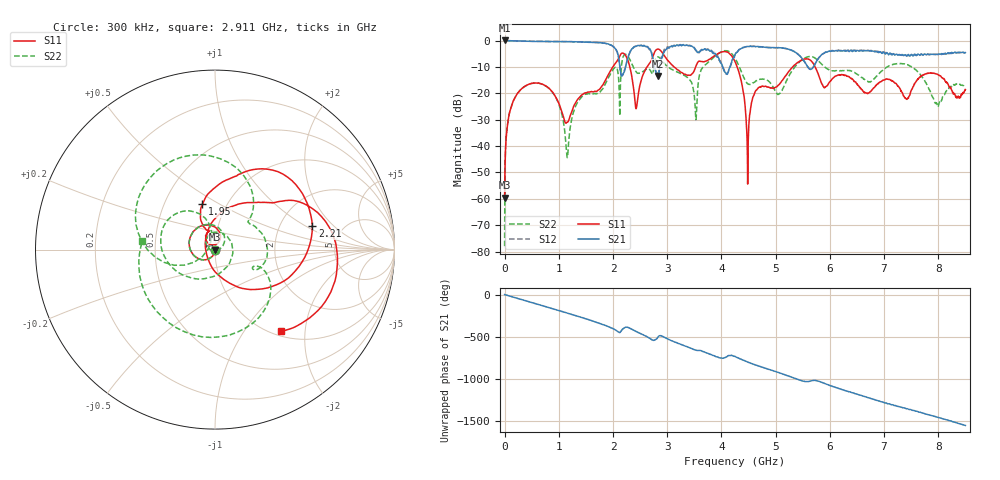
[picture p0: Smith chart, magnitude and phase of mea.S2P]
!Agilent Technologies,E5071B,MY42402595,A.08.01
!Date: Mon Jan 01 22:53:59 2001
!Data & Calibration Information:
!Freq	S11:SOLT2(ON)	S21:SOLT2(ON)	S12:SOLT2(ON)	S22:SOLT2(ON)
# Hz S dB R 50
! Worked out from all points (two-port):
!   1601 points, 300 kHz to 8.5 GHz, reference 50 ohm
!   highest |S21| = 0.04 dB at 300 kHz (marker M1); lowest = -13.5 dB at 2.821 GHz (marker M2)
!   |S21| within 3 dB of the highest: start of sweep to 2.038 GHz; 4.368 GHz to 5.173 GHz (804.4 MHz wide, 16.9 % of centre)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
!   lowest |S11| = -59.6 dB at 300 kHz (marker M3), VSWR 1.00, Z = 50 - j0.101 ohm
!   |S11| at or under -10 dB: start of sweep to 1.997 GHz; 4.291 GHz to 5.313 GHz (1.022 GHz wide, 21.3 % of centre); 5.728 GHz to end of sweep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
!   |S22| runs from -78.0 to -3.8 dB; largest |S21 - S12| = 0.071
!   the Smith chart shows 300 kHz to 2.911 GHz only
!   S11 on the Smith chart (normalised r, x): 300 kHz: 1.00, -0.00; 1.95 GHz: 0.77, +0.42; 2.21 GHz: 3.04, +1.15; 2.911 GHz: 1.09, -1.50
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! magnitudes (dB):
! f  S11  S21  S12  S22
! 300 kHz  -59.6  0.0  0.0  -78.0
! 64.05 MHz  -30.4  0.0  0.0  -30.4
! 250 MHz  -19.7  -0.1  -0.1  -19.8
! 845 MHz  -18.6  -0.4  -0.4  -18.7
! 1.153 GHz  -30.9  -0.4  -0.4  -44.3
! 1.419 GHz  -20.7  -0.5  -0.6  -21.4
! 1.95 GHz  -11.6  -1.6  -1.7  -12.7
! 2.21 GHz  -5.1  -11.7  -11.2  -5.4
! 2.433 GHz  -25.3  -2.1  -2.0  -12.0
! 2.821 GHz  -3.3  -13.5  -12.4  -6.2
! 2.837 GHz  -3.2  -12.7  -12.2  -6.2
! 2.911 GHz  -4.7  -5.7  -6.3  -7.8
! 3.522 GHz  -10.1  -3.4  -3.7  -28.2
! 3.676 GHz  -8.1  -3.3  -3.2  -9.7
! 4.25 GHz  -7.9  -5.3  -5.5  -6.7
! 4.489 GHz  -45.0  -2.2  -2.3  -16.5
! 4.665 GHz  -18.4  -2.2  -2.3  -15.1
! 5.068 GHz  -16.6  -2.7  -2.7  -20.1
! 5.669 GHz  -8.0  -10.8  -10.7  -6.1
! 7.087 GHz  -14.7  -5.3  -4.8  -9.6
! 7.974 GHz  -12.7  -5.2  -5.2  -23.8
! 8.5 GHz  -18.6  -4.6  -4.7  -17.8
